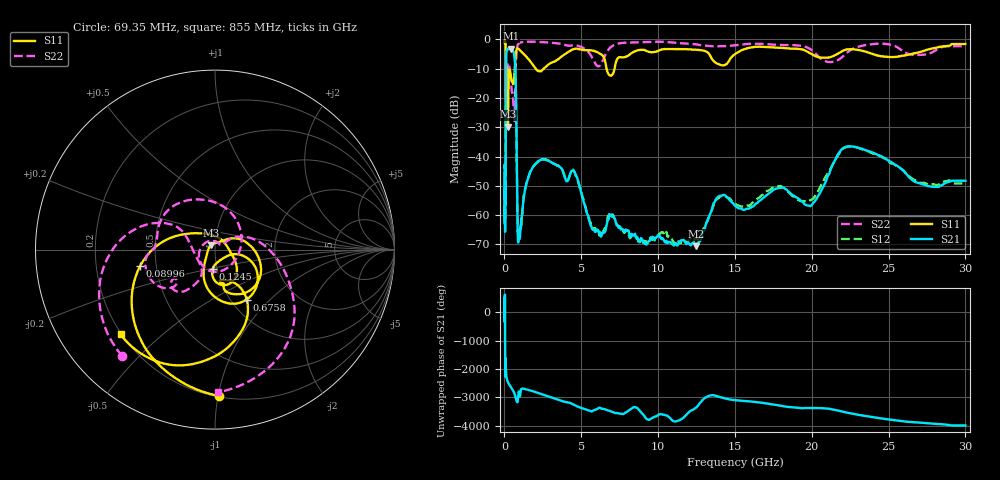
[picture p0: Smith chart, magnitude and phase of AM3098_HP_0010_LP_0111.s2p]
! Date/Time: Thu, Feb 28, 2019 8:33 AM
! Network Analyzer: Agilent Technologies E8364B Rev: A.07.50.67
! Sweep from 0.010 to 30.000 GHz, 1601 Points, Sweep Type: LOG
! Power Supply: 5.022 V, 0.002 A
# Hz S DB R 50
!freq MagS11 AngS11 MagS21 AngS21 MagS12 AngS12 MagS22 AngS22
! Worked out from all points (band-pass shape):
!   1601 points, 10 MHz to 30 GHz, reference 50 ohm
!   highest |S21| = -3.10 dB at 411.8 MHz (marker M1); lowest = -70.6 dB at 12.5 GHz (marker M2)
!   |S21| within 3 dB of the highest: 106.2 MHz to 660.4 MHz (554.2 MHz wide, 145 % of centre)
!   lowest |S11| = -29.8 dB at 227 MHz (marker M3), VSWR 1.07, Z = 47.9 + j2.38 ohm
!   |S11| at or under -10 dB: 176 MHz to 671.3 MHz (495.3 MHz wide, 117 % of centre); 2.042 GHz to 2.554 GHz (512.1 MHz wide, 22.3 % of centre); 6.645 GHz to 7.165 GHz (520.6 MHz wide, 7.54 % of centre)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
!   |S22| runs from -28.3 to -0.5 dB; largest |S21 - S12| = 0.011
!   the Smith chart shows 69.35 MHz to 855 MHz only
!   S11 on the Smith chart (normalised r, x): 69.35 MHz: 0.21, -1.00; 89.96 MHz: 0.41, -0.09; 124.5 MHz: 0.95, -0.20; 675.8 MHz: 1.18, -0.74; 855 MHz: 0.20, -0.37
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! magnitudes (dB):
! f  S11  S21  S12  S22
! 10 MHz  -0.3  -43.7  -45.9  -0.5
! 38.04 MHz  -0.5  -63.5  -59.7  -0.9
! 69.35 MHz  -1.8  -54.1  -50.4  -2.1
! 89.96 MHz  -7.4  -20.5  -20.5  -8.5
! 99.92 MHz  -23.7  -8.1  -8.1  -17.0
! 124.5 MHz  -19.5  -4.4  -4.4  -10.5
! 144.7 MHz  -13.6  -3.7  -3.7  -10.3
! 185.8 MHz  -11.3  -3.6  -3.5  -8.0
! 227 MHz  -29.8  -3.2  -3.2  -9.4
! 411.8 MHz  -12.3  -3.1  -3.1  -12.8
! 550.5 MHz  -15.1  -3.8  -3.7  -19.3
! 675.8 MHz  -9.6  -7.0  -7.0  -22.6
! 747 MHz  -4.8  -17.9  -17.9  -8.0
! 855 MHz  -3.0  -63.3  -62.2  -2.0
! 2.084 GHz  -10.3  -42.3  -42.1  -0.8
! 4.48 GHz  -3.3  -44.8  -44.6  -2.0
! 7.926 GHz  -5.9  -65.4  -65.5  -1.1
! 12.5 GHz  -3.5  -70.6  -68.4  -1.7
! 14.09 GHz  -8.7  -53.5  -53.6  -2.3
! 19.9 GHz  -4.7  -57.0  -54.9  -3.3
! 22.56 GHz  -3.3  -36.5  -36.7  -3.5
! 30 GHz  -1.6  -48.3  -49.2  -2.3
